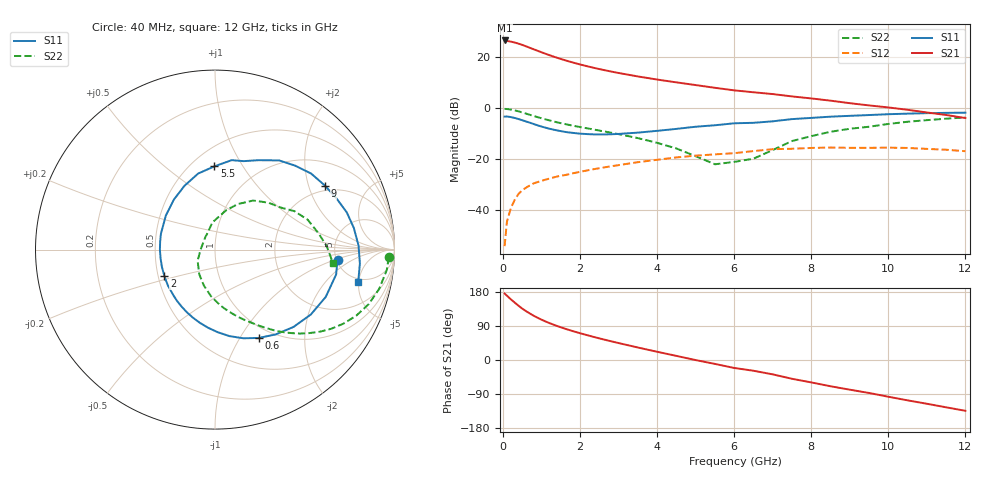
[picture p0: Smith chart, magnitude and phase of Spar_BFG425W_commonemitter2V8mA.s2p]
! Filename: 28bfg425.001
! BFG425W Field C1
! V1=8.411E-001V,V2=2.000E+000V, I1=1.071E-004A, I2=8.000E-003A
# GHz  S  MA  R 50
!  S11  S21  S12  S22
!Freq(GHz)  Mag  Ang  Mag  Ang  Mag  Ang  Mag  Ang
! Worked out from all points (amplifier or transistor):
!   44 points, 40 MHz to 12 GHz, reference 50 ohm
!   highest |S21| = 26.5 dB at 40 MHz (marker M1)
!   |S21| within 3 dB of that: start of sweep to 716.9 MHz
!   unconditionally stable (mu >= 1): 2.063 GHz to end of sweep
!   at 700 MHz: K = 0.46, MSG = 26.9 dB, |S12| = -30.2 dB
!   at 2.4 GHz: K = 1.07, MAG = 18.0 dB, |S12| = -23.7 dB
!   at 12 GHz: K = 1.41, MAG = 2.7 dB, |S12| = -16.8 dB
!   S11 on the Smith chart (normalised r, x): 40 MHz: 5.11, -1.09; 600 MHz: 0.86, -1.21; 2 GHz: 0.54, -0.18; 5.5 GHz: 0.64, +0.76; 9 GHz: 1.80, +2.58; 12 GHz: 4.54, -4.92
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0.04  0.685 -4.7  21.15 175.3  0.002 81.7  0.969 -2.5
0.2  0.671 -23.1  20.09 160.3  0.011 77.5  0.941 -13.4
0.3  0.645 -34.1  19.28 151.7  0.016 72.3  0.909 -19.5
0.4  0.614 -44.6  18.32 143.3  0.021 67.2  0.869 -25.1
0.5  0.581 -54.5  17.3 135.5  0.025 63.0  0.826 -30.0
0.6  0.549 -63.7  16.19 128.6  0.028 59.5  0.783 -34.3
0.8  0.489 -80.4  14.17 116.6  0.034 53.8  0.702 -41.5
0.9  0.461 -88.0  13.25 111.2  0.036 51.7  0.667 -44.5
1.2  0.398 -108.2  10.93 97.6  0.042 46.8  0.578 -52.0
1.4  0.368 -120.4  9.715 89.9  0.046 44.7  0.53 -56.1
1.6  0.345 -131.9  8.713 82.9  0.049 42.8  0.491 -59.8
2  0.318 -152.6  7.17 70.6  0.057 39.7  0.428 -66.8
2.2  0.311 -162.2  6.572 65.0  0.061 38.1  0.402 -70.3
3  0.314 163.5  4.882 44.7  0.077 30.9  0.311 -84.7
3.5  0.333 145.4  4.182 33.0  0.088 25.5  0.26 -95.0
4.5  0.394 115.6  3.202 10.8  0.109 12.6  0.163 -122.6
5.5  0.464 90.4  2.505 -10.3  0.125 -1.8  0.08 179.5
6.5  0.518 72.1  2.05 -28.4  0.145 -12.7  0.103 113.0
8.5  0.683 38.3  1.405 -69.3  0.17 -48.9  0.346 52.2
9  0.709 30.1  1.254 -78.4  0.168 -57.0  0.396 41.4
10.5  0.783 8.8  0.931 -106.5  0.167 -83.6  0.543 17.8
12  0.818 -12.7  0.642 -134.0  0.144 -113.4  0.661 -6.5
